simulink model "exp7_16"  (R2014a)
settings: Solver=ode45  StartTime=0.0  StopTime=10.0  RelTol=1e-3
libraries: commdigbbndpm3 x2, commchan3 x1, commsink2 x1, commrandsrc2 x1

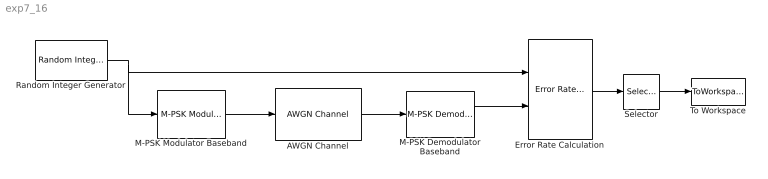
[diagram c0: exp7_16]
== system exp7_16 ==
  AWGN Channel : commchan3/AWGN Channel  InputProcessing=Columns as channels (frame based)  seed=67  noiseMode="Signal to noise ratio  (Eb/No)"  EbNodB=10  EsNodB=10  SNRdB=10  bitsPerSym=1  Ps=1  Tsym=1  variance=1
  Error Rate Calculation : commsink2/Error Rate Calculation  N=0  st_delay=0  cp_mode=Entire frame  subframe=[]  PMode=Port  WsName=ErrorVec  RsMode2=off  stop=off  numErr=100  maxBits=1e6
  M-PSK Demodulator Baseband : commdigbbndpm3/M-PSK Demodulator Baseband  M=8  Ph=pi/8  Dec=Gray  Mapping=[0:7]  OutType=Integer  DecType=Hard decision  VarSource=Dialog  Variance=1  outDtype1=Inherit via internal rule  outDtype2=Inherit via internal rule  derotateFactorWordLen=16
  M-PSK Modulator Baseband : commdigbbndpm3/M-PSK Modulator Baseband  M=8  InType=Integer  Enc=Gray  Mapping=[0:7]  Ph=pi/8  outDtype=double  outWordLen=16  outUDDataType=sfix(16)  outFracLenMode=Best precision  outFracLen=15
  Random Integer Generator : commrandsrc2/Random Integer Generator  mul=8  seed=37  Ts=1  frameBased=off  sampPerFrame=1  orient=off  outDataType=double
  Selector : Selector  InputPortWidth=3  Indices=[1]
  To Workspace : ToWorkspace  VariableName=simout  SaveFormat=Timeseries  SampleTime=-1
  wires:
  Random Integer Generator/1 -> M-PSK Modulator Baseband/1, Error Rate Calculation/1
  M-PSK Modulator Baseband/1 -> AWGN Channel/1
  AWGN Channel/1 -> M-PSK Demodulator Baseband/1
  M-PSK Demodulator Baseband/1 -> Error Rate Calculation/2
  Error Rate Calculation/1 -> Selector/1
  Selector/1 -> To Workspace/1
